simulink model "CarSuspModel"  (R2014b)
settings: Solver=ode45  StartTime=0.0  StopTime=5.0  RelTol=1e-3
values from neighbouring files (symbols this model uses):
  A = [0 1 0 0    [CarSuspData.m]
  B = [0 1/m1 0 (1/m1)+(1/m2)    [CarSuspData.m]
  C = [0 0 1 0]    [CarSuspData.m]    (also in GantryData.m)

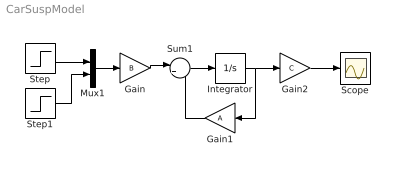
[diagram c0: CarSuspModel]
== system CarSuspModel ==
  Gain : Gain  Gain=B  Multiplication=Matrix(K*u) (u vector)
  Gain1 : Gain  Gain=A  Multiplication=Matrix(K*u) (u vector)
  Gain2 : Gain  Gain=C  Multiplication=Matrix(K*u) (u vector)
  Integrator : Integrator
  Mux1 : Mux  Inputs=2
  Scope : Scope
  Step : Step  SampleTime=0
  Step1 : Step  After=0  SampleTime=0
  Sum1 : Sum  Inputs=|++
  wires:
  Integrator/1 -> Gain2/1, Gain1/1
  Gain/1 -> Sum1/1
  Gain1/1 -> Sum1/2
  Sum1/1 -> Integrator/1
  Mux1/1 -> Gain/1
  Gain2/1 -> Scope/1
  Step/1 -> Mux1/1
  Step1/1 -> Mux1/2
